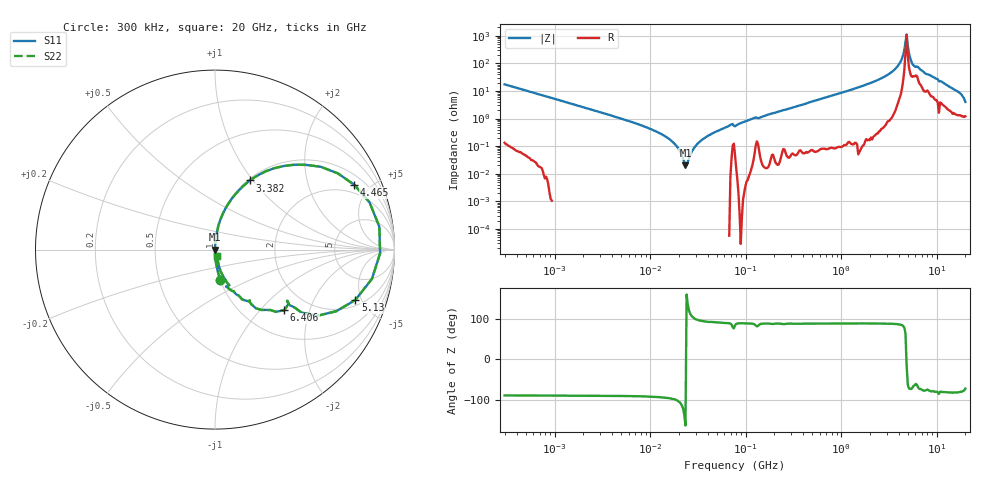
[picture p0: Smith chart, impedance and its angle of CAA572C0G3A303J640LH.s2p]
! S-Parameter Data Generated by TDK Corporation
! Copyright(C) 2022 TDK Corporation.
! All Rights Reserved.
! TDK P/N: CAA572C0G3A303J640LH (Multilayer Ceramic Chip Capacitor)
! Property: C=30nF
! Size(LxWxT): 6x5.6x6.4mm
! Model Type: s2p (Touchstone File Format Version 1.0)
! Frequency: DC=Yes Start=0.3MHz Stop=20000MHz 402points Log-sweep
! Model Generated on Apr. 15, 2022
! Port Assignments:
!  1 ---| |--- 2
! Applicable Conditions:
!  Temperature = 25 degC
!  DC Bias Voltage = 0 V
!  Small Signal Operation
! Terms and conditions regarding TDK Simulation Models
! (1)This simulation model is being provided solely for informational purposes. Please refer to the specifications of the products in terms of detailed characteristics of such products.
! (2)In no event shall TDK Corporation of any of its subsidiaries be liable for any loss or damage arising, directly or indirectly,
!  From any information contained in this simulation model, including, but not limited to loss or damages arising from any inaccuracies, omissions or errors in connection with such information.
! (3)Any and all copyrights on this simulation model are owned by TDK Corporation.
!  Duplication or redistribution of this simulation model without prior written permission from TDK Corporation is prohibited.
! (4)This simulation model is subject to any modification or change without any prior notice.
! (5)Neither TDK Corporation nor any of its subsidiaries shall make any warranty, express or implied,
!  Including but not limited to the correctness, implied warranties of merchantability and fitness for a particular purpose with respect to this simulation models.
! (6)The use of this simulation model shall be deemed to have consented to the terms and conditions hereof.
# Hz S MA R 50
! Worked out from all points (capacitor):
!   401 points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, 300 kHz to 20 GHz, reference 50 ohm
!   read as one part in series: C = 30.7 nF near 317.1 kHz
!   lowest |Z| = 20.2 mohm at 23.47 MHz (marker M1)
!   series resonance near 23.77 MHz, so ESL is about 1.5 nH
!   S11 on the Smith chart (normalised r, x): 300 kHz: 1.00, -0.35; 3.382 GHz: 1.02, +0.97; 4.465 GHz: 1.48, +4.01; 5.13 GHz: 2.45, -4.44; 6.406 GHz: 1.50, -1.37; 20 GHz: 1.02, -0.08
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300000  0.1702 -79.8  0.9841 9.8  0.9841 9.8  0.1702 -79.8
1928084  0.0267 -88.8  0.9998 1.5  0.9998 1.5  0.0267 -88.8
1.239169e7  0.003035 -93.7  1 0.2  1 0.2  0.003035 -93.7
1.827963e7  0.001163 -99.7  1 0.1  1 0.1  0.001163 -99.7
2.346959e7  0.0002019 -164.3  1 0.0  1 0.0  0.0002019 -164.3
2.930783e7  0.0009242 101.5  1 -0.1  1 -0.1  0.0009242 101.5
3.559607e7  0.001777 95.3  1 -0.1  1 -0.1  0.001777 95.3
6.931649e7  0.005807 88.9  0.9999 -0.3  0.9999 -0.3  0.005807 88.9
7.964076e7  0.005623 88.0  0.9998 -0.3  0.9998 -0.3  0.005623 88.0
4.978292e8  0.04123 86.6  0.9984 -2.4  0.9984 -2.4  0.04123 86.6
1.643049e9  0.1466 81.2  0.9883 -8.4  0.9883 -8.4  0.1466 81.2
3.199522e9  0.385 66.2  0.9154 -22.6  0.9154 -22.6  0.385 66.2
3.382241e9  0.432 63.2  0.8926 -25.6  0.8926 -25.6  0.432 63.2
4.10793e9  0.6927 42.9  0.6824 -43.8  0.6824 -43.8  0.6927 42.9
4.464803e9  0.8562 24.9  0.4244 -58.2  0.4244 -58.2  0.8562 24.9
4.719781e9  0.9246 7.9  0.1528 -56.5  0.1528 -56.5  0.9246 7.9
5.129809e9  0.8309 -19.7  0.3554 52.2  0.3554 52.2  0.8309 -19.7
5.575457e9  0.5957 -36.0  0.6255 34.1  0.6255 34.1  0.5957 -36.0
6.405888e9  0.5125 -41.2  0.7013 28.8  0.7013 28.8  0.5125 -41.2
9.989315e9  0.2545 -65.7  0.925 14.5  0.925 14.5  0.2545 -65.7
1.601592e10  0.1018 -76.6  0.9814 5.8  0.9814 5.8  0.1018 -76.6
2e10  0.03939 -70.3  0.9874 2.2  0.9874 2.2  0.03939 -70.3
